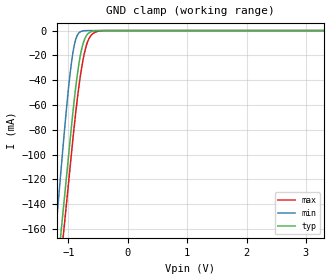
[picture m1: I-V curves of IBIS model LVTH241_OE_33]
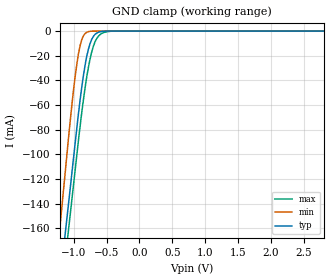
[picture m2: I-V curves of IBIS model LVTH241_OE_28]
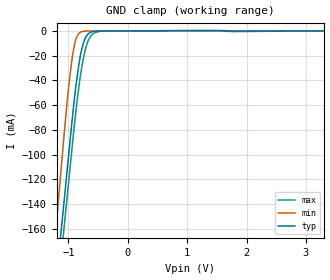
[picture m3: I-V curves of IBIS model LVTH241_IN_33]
| TEXAS INSTRUMENTS INCORPORATED
| Standard Linear and Logic Group
| IBIS Model of SN74LVTH241
| 3.3-V ABT OCTAL BUFFERS/DRIVERS WITH 3-STATE OUTPUTS
| This file contains package information for the following:
|  SSOP 20-pin (DB) package as [Component] LVTH241_DB
|  SOIC 20-pin (DW) package as [Component] LVTH241_DW
|  SOP 20-pin (NS) package as [Component] LVTH241_NS
|  TSSOP 20-pin (PW) package as [Component] LVTH241_PW
| This device can be powered at the following Vccs:
|  3.3 volt Vcc
|  2.8 volt Vcc
| This file provides unique models under the [Model Selector] for each Vcc.
| For operation at a specific Vcc, select the appropriate model after each
| [Model Selector] keyword.
[IBIS Ver]   3.2
[Comment char]  |_char
[File Name]   sn74lvth241.ibs
[File Rev]   1.1 | a_die
[Date]   June 17, 2002
[Source]   Data created from TI-SPICE simulations at TI-SLL.
[Notes]   The following is an IBIS list for the LVTH241A_DL.
   Please contact sllibis@ti.com with questions and
   comments concerning SLL IBIS models.
   - Due to presence of BUS HOLD at input, GND-CLAMP curves
   have non-monotonic warnings.
   - Non-monotonic data in pullup as the device is
   overvoltage tolerant.
   - We omitted Power_Clamp table data from the input models,
   since there is no power clamp diode at input.
[Disclaimer] Property of Texas Instruments Incorporated.  Unauthorized
   reproduction and/or distribution is strictly prohibited.
   This product is protected under copyright law.
   Created  2002, (C) Copyright  2002, Texas Instruments
   Incorporated, All Rights Reserved
   UNLESS THERE IS A SIGNED, WRITTEN AGREEMENT TO THE
   CONTRARY, TEXAS INSTRUMENTS (TI) IS PROVIDING THE IBIS
   MODELS  AND WITHOUT ANY WARRANTY, EXPRESSED OR
   IMPLIED.  TI assumes no liability for:
   1) the accuracy of the IBIS models provided to your
   company;
   2) the proper functioning of these IBIS Models in your
   design or for any resulting applications; or
   3) infringement of patents, copyrights or intellectual
   property rights resulting from your use of these IBIS
   models.
   TI provides IBIS Models as a service to our customers.
   You and your company shall not distribute, sell or give
   these models to anyone else without prior written
   permission from TI.
   TI reserves the right to make changes to our products or
   to discontinue any semiconductor product or service
   without notice, and advises our customers to obtain the
   latest version of relevant information to verify, before
   placing orders, that the information being relied on is
   current.
   Please be aware that your receipt and use of the IBIS
   information provided shall serve as acceptance of these
   terms and conditions.  If you do not accept these terms,
   you should return or destroy the IBIS models and any
   other accompanying information immediately.
| Component LVTH241_DB 20-pin SSOP
[Component]   LVTH241_DB
[Manufacturer]   Texas Instruments, Inc.
[Package]
|   typ   min   max
R_pkg   4.000e-02   3.500e-02   5.100e-02
L_pkg   3.495e-09   3.035e-09   4.314e-09
C_pkg   4.200e-13   3.460e-13   5.020e-13
[Pin]   signal_name   model_name   R_pin   L_pin   C_pin
1   1NOE   LVTH241_OE   4.900e-02   4.310e-09   5.020e-13
2   1A1   LVTH241_IN   4.800e-02   3.903e-09   4.870e-13
3   2Y4   LVTH241_OUT   3.500e-02   3.189e-09   3.960e-13
4   1A2   LVTH241_IN   3.500e-02   3.036e-09   3.470e-13
5   2Y3   LVTH241_OUT   3.500e-02   3.035e-09   3.670e-13
6   1A3   LVTH241_IN   3.500e-02   3.035e-09   3.670e-13
7   2Y2   LVTH241_OUT   3.500e-02   3.036e-09   3.470e-13
8   1A4   LVTH241_IN   3.500e-02   3.189e-09   3.970e-13
9   2Y1   LVTH241_OUT   4.700e-02   3.899e-09   4.880e-13
10   GND   GND   5.100e-02   4.314e-09   5.000e-13
11   2A1   LVTH241_IN   5.100e-02   4.314e-09   5.000e-13
12   1Y4   LVTH241_OUT   4.700e-02   3.899e-09   4.880e-13
13   2A2   LVTH241_IN   3.500e-02   3.189e-09   3.970e-13
14   1Y3   LVTH241_OUT   3.500e-02   3.036e-09   3.460e-13
15   2A3   LVTH241_IN   3.500e-02   3.035e-09   3.670e-13
16   1Y2   LVTH241_OUT   3.500e-02   3.035e-09   3.670e-13
17   2A4   LVTH241_IN   3.500e-02   3.036e-09   3.460e-13
18   1Y1   LVTH241_OUT   3.500e-02   3.189e-09   3.970e-13
19   2OE   LVTH241_OE   4.700e-02   3.899e-09   4.880e-13
20   VCC   POWER   5.100e-02   4.314e-09   5.020e-13
| Component LVTH241_DW 20-pin SOIC
[Component]   LVTH241_DW
[Manufacturer]   Texas Instruments, Inc.
[Package]
|   typ   min   max
R_pkg   3.800e-02   3.300e-02   4.500e-02
L_pkg   5.012e-09   4.110e-09   6.349e-09
C_pkg   7.170e-13   5.300e-13   8.680e-13
[Pin]   signal_name   model_name   R_pin   L_pin   C_pin
1   1NOE   LVTH241_OE   4.200e-02   6.336e-09   8.650e-13
2   1A1   LVTH241_IN   4.300e-02   5.542e-09   8.670e-13
3   2Y4   LVTH241_OUT   3.400e-02   4.714e-09   7.320e-13
4   1A2   LVTH241_IN   3.400e-02   4.377e-09   5.910e-13
5   2Y3   LVTH241_OUT   3.600e-02   4.130e-09   5.330e-13
6   1A3   LVTH241_IN   3.500e-02   4.111e-09   5.300e-13
7   2Y2   LVTH241_OUT   3.400e-02   4.284e-09   5.830e-13
8   1A4   LVTH241_IN   3.400e-02   4.634e-09   7.260e-13
9   2Y1   LVTH241_OUT   4.000e-02   5.518e-09   8.650e-13
10   GND   GND   4.300e-02   6.349e-09   8.660e-13
11   2A1   LVTH241_IN   4.100e-02   6.281e-09   8.610e-13
12   1Y4   LVTH241_OUT   4.500e-02   5.561e-09   8.680e-13
13   2A2   LVTH241_IN   3.300e-02   4.778e-09   7.420e-13
14   1Y3   LVTH241_OUT   3.500e-02   4.414e-09   5.960e-13
15   2A3   LVTH241_IN   3.500e-02   4.110e-09   5.330e-13
16   1Y2   LVTH241_OUT   3.600e-02   4.130e-09   5.330e-13
17   2A4   LVTH241_IN   3.400e-02   4.377e-09   5.910e-13
18   1Y1   LVTH241_OUT   3.400e-02   4.714e-09   7.310e-13
19   2OE   LVTH241_OE   4.300e-02   5.569e-09   8.680e-13
20   VCC   POWER   4.200e-02   6.308e-09   8.640e-13
| Component LVTH241_NS 20-pin SOP
[Component]   LVTH241_NS
[Manufacturer]   Texas Instruments, Inc.
[Package]
|   typ   min   max
R_pkg   4.400e-02   2.900e-02   5.800e-02
L_pkg   3.666e-09   2.317e-09   5.115e-09
C_pkg   5.480e-13   3.160e-13   7.250e-13
[Pin]   signal_name   model_name   R_pin   L_pin   C_pin
1   1NOE   LVTH241_OE   5.800e-02   5.115e-09   7.250e-13
2   1A1   LVTH241_IN   5.300e-02   4.591e-09   7.240e-13
3   2Y4   LVTH241_OUT   4.900e-02   3.754e-09   5.720e-13
4   1A2   LVTH241_IN   2.900e-02   2.549e-09   3.880e-13
5   2Y3   LVTH241_OUT   3.100e-02   2.317e-09   3.160e-13
6   1A3   LVTH241_IN   3.100e-02   2.317e-09   3.160e-13
7   2Y2   LVTH241_OUT   2.900e-02   2.556e-09   3.990e-13
8   1A4   LVTH241_IN   4.900e-02   3.754e-09   5.790e-13
9   2Y1   LVTH241_OUT   5.300e-02   4.591e-09   7.240e-13
10   GND   GND   5.800e-02   5.115e-09   7.250e-13
11   2A1   LVTH241_IN   5.800e-02   5.115e-09   7.250e-13
12   1Y4   LVTH241_OUT   5.300e-02   4.591e-09   7.240e-13
13   2A2   LVTH241_IN   4.900e-02   3.754e-09   5.790e-13
14   1Y3   LVTH241_OUT   2.900e-02   2.557e-09   3.990e-13
15   2A3   LVTH241_IN   3.100e-02   2.317e-09   3.160e-13
16   1Y2   LVTH241_OUT   3.100e-02   2.317e-09   3.160e-13
17   2A4   LVTH241_IN   2.900e-02   2.557e-09   3.990e-13
18   1Y1   LVTH241_OUT   4.900e-02   3.754e-09   5.790e-13
19   2OE   LVTH241_OE   5.300e-02   4.591e-09   7.240e-13
20   VCC   POWER   5.800e-02   5.115e-09   7.250e-13
| Component LVTH241_PW 20-pin TSSOP
[Component]   LVTH241_PW
[Manufacturer]   Texas Instruments, Inc.
[Package]
|   typ   min   max
R_pkg   5.000e-02   4.200e-02   6.000e-02
L_pkg   2.802e-09   2.248e-09   3.553e-09
C_pkg   3.170e-13   2.020e-13   4.430e-13
[Pin]   signal_name   model_name   R_pin   L_pin   C_pin
1   1NOE   LVTH241_OE   5.500e-02   3.461e-09   4.400e-13
2   1A1   LVTH241_IN   5.500e-02   3.150e-09   4.010e-13
3   2Y4   LVTH241_OUT   4.200e-02   2.619e-09   3.020e-13
4   1A2   LVTH241_IN   4.500e-02   2.273e-09   2.020e-13
5   2Y3   LVTH241_OUT   4.500e-02   2.248e-09   2.240e-13
6   1A3   LVTH241_IN   4.500e-02   2.273e-09   2.260e-13
7   2Y2   LVTH241_OUT   4.400e-02   2.323e-09   2.050e-13
8   1A4   LVTH241_IN   4.600e-02   2.704e-09   3.070e-13
9   2Y1   LVTH241_OUT   6.000e-02   3.265e-09   4.110e-13
10   GND   GND   5.700e-02   3.506e-09   4.360e-13
11   2A1   LVTH241_IN   5.800e-02   3.553e-09   4.370e-13
12   1Y4   LVTH241_OUT   5.800e-02   3.193e-09   4.050e-13
13   2A2   LVTH241_IN   4.200e-02   2.704e-09   3.110e-13
14   1Y3   LVTH241_OUT   4.600e-02   2.392e-09   2.100e-13
15   2A3   LVTH241_IN   4.700e-02   2.334e-09   2.290e-13
16   1Y2   LVTH241_OUT   4.700e-02   2.300e-09   2.270e-13
17   2A4   LVTH241_IN   4.700e-02   2.349e-09   2.070e-13
18   1Y1   LVTH241_OUT   4.500e-02   2.677e-09   3.060e-13
19   2OE   LVTH241_OE   6.000e-02   3.235e-09   4.060e-13
20   VCC   POWER   5.600e-02   3.487e-09   4.430e-13
| Model LVTH241_OE
[Model Selector]   LVTH241_OE
LVTH241_OE_33   3.3 volt Vcc
LVTH241_OE_28   2.8 volt Vcc
| Model LVTH241_IN
[Model Selector]   LVTH241_IN
LVTH241_IN_33   3.3 volt Vcc
LVTH241_IN_28   2.8 volt Vcc
| Model LVTH241_OUT
[Model Selector]   LVTH241_OUT
LVTH241_OUT_33   3.3 volt Vcc
LVTH241_OUT_28   2.8 volt Vcc
| Models and submodels in the file (6): LVTH241_OE_33 (Input), LVTH241_OE_28 (Input), LVTH241_IN_33 (Input), LVTH241_IN_28 (Input), LVTH241_OUT_33 (3-state), LVTH241_OUT_28 (3-state)
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[Model]   LVTH241_OE_33
Model_type  Input
Vinl = 0.8
Vinh = 2.34
| variable   typ   min   max
C_comp   4.05pF   3.22pF   5.48pF
[Temperature Range]   40   -40   100
| Ambient temperature   25   -40   85
[Voltage range]   3.3   3   3.6
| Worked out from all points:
|   GND clamp passes 1 mA (typ) near -0.62 V on its own axis
[GND Clamp]
| LVTH241_OE_33
|   Voltage   I(typ)   I(min)   I(max)
-5.5V     -2.407A    -2.649A    -2.406A
-1.22V    -209.3mA   -166mA     -230mA
-1.205V   -202mA     -157.6mA   -222.8mA
-1.125V   -163.1mA   -113mA     -184.2mA
-1.075V   -138.8mA   -85.25mA   -160.1mA
-975mV    -90.17mA   -36.12mA   -112mA
-900mV    -55.28mA   -11.44mA   -76.47mA
-825mV    -27.42mA   -1.98mA    -45.67mA
-775mV    -14.64mA   -464.8uA   -29.41mA
-650mV    -1.684mA   -2.076uA   -6.132mA
-395mV    -1.224uA   -43.32pA   -35.77uA
3.3V      16.15pA    8.657pA    1.272nA
[Model]   LVTH241_OE_28
Model_type  Input
Vinl = 0.8
Vinh = 2.0
| variable   typ   min   max
C_comp   4.08pF   3.31pF   5.47pF
[Temperature Range]   40   -40   100
| Ambient temperature   25   -40   85
[Voltage range]   2.8   2.7   2.9
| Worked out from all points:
|   GND clamp passes 1 mA (typ) near -0.62 V on its own axis
[GND Clamp]
| LVTH241_OE_28
|   Voltage   I(typ)   I(min)   I(max)
-5.5V     -2.407A    -2.649A    -2.406A
-1.22V    -209.3mA   -166mA     -230mA
-1.205V   -202mA     -157.6mA   -222.8mA
-1.125V   -163.1mA   -113mA     -184.2mA
-1.075V   -138.8mA   -85.25mA   -160.1mA
-975mV    -90.17mA   -36.12mA   -112mA
-900mV    -55.28mA   -11.44mA   -76.47mA
-800mV    -20.27mA   -984.6uA   -36.91mA
-675mV    -2.699mA   -6.758uA   -8.728mA
-575mV    -336.8uA   -57.38nA   -1.991mA
-425mV    -3.297uA   -110.8pA   -102.1uA
2.8V      13.7pA     7.338pA    757.3pA
[Model]   LVTH241_IN_33
Model_type  Input
Vinl = 0.8
Vinh = 2.34
| variable   typ   min   max
C_comp   3.84pF   3.07pF   5.25pF
[Temperature Range]   40   -40   100
| Ambient temperature   25   -40   85
[Voltage range]   3.3   3   3.6
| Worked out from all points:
|   GND clamp passes 1 mA (typ) near -0.62 V on its own axis
[GND Clamp]
| LVTH241_IN_33
|   Voltage   I(typ)   I(min)   I(max)
-5.5V     -2.408A    -2.65A     -2.407A
-1.22V    -209.4mA   -166.2mA   -230.2mA
-1.19V    -194.8mA   -149.4mA   -215.7mA
-1.125V   -163.2mA   -113.2mA   -184.4mA
-1.075V   -138.9mA   -85.44mA   -160.3mA
-975mV    -90.33mA   -36.32mA   -112.1mA
-900mV    -55.43mA   -11.64mA   -76.61mA
-825mV    -27.57mA   -2.159mA   -45.81mA
-775mV    -14.79mA   -632.4uA   -29.53mA
-650mV    -1.834mA   -141.2uA   -6.249mA
-405mV    -96.3uA    -83.9uA    -154.2uA
3.3V      19.45pA    12.56pA    -1.138uA
